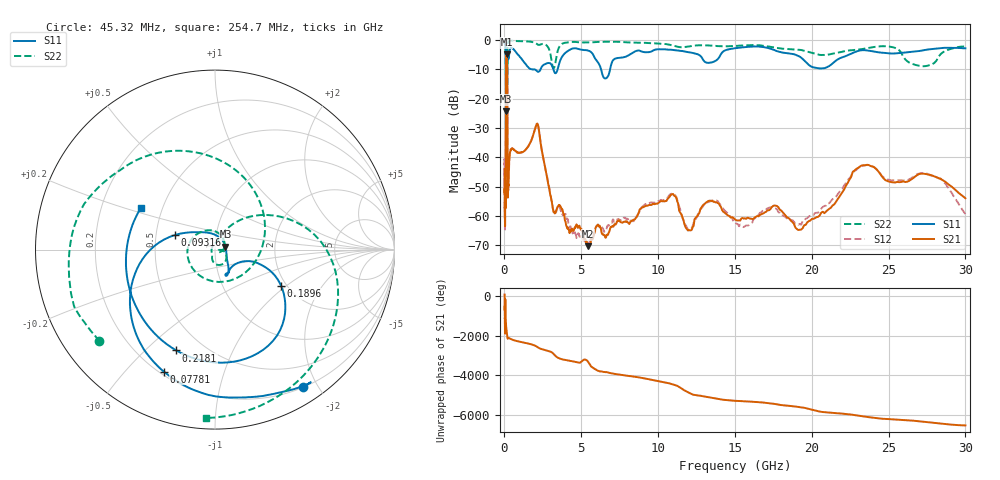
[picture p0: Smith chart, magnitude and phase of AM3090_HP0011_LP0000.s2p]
! Date/Time: Thu, Feb 28, 2019 1:56 PM
! Network Analyzer: Agilent Technologies E8364B Rev: A.07.50.67
! Sweep from 0.010 to 30.000 GHz, 1601 Points, Sweep Type: LOG
! Power Supply: 5.022 V, 0.002 A
# Hz S DB R 50
!freq MagS11 AngS11 MagS21 AngS21 MagS12 AngS12 MagS22 AngS22
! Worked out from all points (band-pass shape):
!   1601 points, 10 MHz to 30 GHz, reference 50 ohm
!   highest |S21| = -4.85 dB at 133.6 MHz (marker M1); lowest = -70.4 dB at 5.446 GHz (marker M2)
!   |S21| within 3 dB of the highest: 100.9 MHz to 174.5 MHz (73.56 MHz wide, 53.4 % of centre)
!   lowest |S11| = -24.3 dB at 100.4 MHz (marker M3), VSWR 1.13, Z = 56.2 + j1.89 ohm
!   |S11| at or under -10 dB: 1.808 GHz to 2.35 GHz (542 MHz wide, 26.1 % of centre); 3.186 GHz to 3.459 GHz (273.7 MHz wide, 8.24 % of centre); 6.288 GHz to 6.877 GHz (588.8 MHz wide, 8.94 % of centre)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
!   |S22| runs from -35.7 to -0.1 dB; largest |S21 - S12| = 0.0091
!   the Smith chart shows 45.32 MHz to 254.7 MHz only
!   S11 on the Smith chart (normalised r, x): 45.32 MHz: 0.20, -1.80; 77.81 MHz: 0.22, -0.64; 93.16 MHz: 0.63, +0.11; 189.6 MHz: 1.87, -0.92; 218.1 MHz: 0.36, -0.63; 254.7 MHz: 0.38, +0.23
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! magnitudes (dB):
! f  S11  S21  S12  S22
! 10 MHz  -0.2  -44.0  -40.6  -0.5
! 38.04 MHz  -0.5  -56.9  -60.2  -1.3
! 45.32 MHz  -0.8  -57.5  -53.1  -1.7
! 71.82 MHz  -1.9  -57.0  -51.8  -3.7
! 77.81 MHz  -2.7  -45.3  -46.2  -5.3
! 93.16 MHz  -12.5  -14.1  -14.1  -15.2
! 100.4 MHz  -24.3  -8.0  -8.0  -17.1
! 133.6 MHz  -16.6  -4.9  -4.8  -33.5
! 144.7 MHz  -16.5  -5.0  -4.9  -22.0
! 169.8 MHz  -15.6  -6.9  -6.8  -34.5
! 189.6 MHz  -7.5  -19.1  -19.1  -10.0
! 218.1 MHz  -4.4  -53.8  -52.1  -1.5
! 254.7 MHz  -6.5  -49.7  -50.0  -0.5
! 550.5 MHz  -3.0  -37.1  -37.2  -0.2
! 2.084 GHz  -10.5  -28.8  -28.8  -1.3
! 3.22 GHz  -10.6  -58.8  -58.7  -9.6
! 5.446 GHz  -3.6  -70.4  -69.3  -0.8
! 7.926 GHz  -5.6  -62.1  -60.9  -0.8
! 10.76 GHz  -3.3  -53.4  -52.8  -1.6
! 19.51 GHz  -6.9  -63.2  -61.7  -3.6
! 23.48 GHz  -3.5  -42.8  -42.7  -2.9
! 30 GHz  -2.8  -54.0  -59.4  -2.2
